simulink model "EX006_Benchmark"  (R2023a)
settings: Solver=ode23tb  StartTime=0.0  StopTime=20e3  MaxStep=1e-1  RelTol=1e-4
undefined symbols (not defined in the file or in its folder): anodeSupplyPressure
libraries: component_lib x38, slpidlib x5, simulink x1, base_lib x1

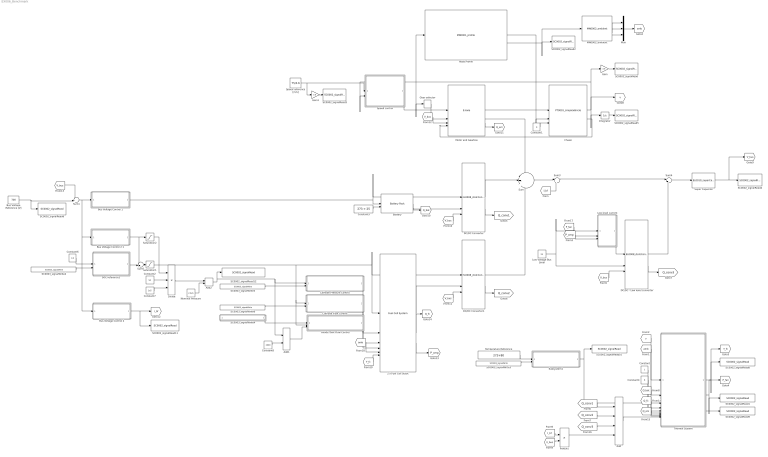
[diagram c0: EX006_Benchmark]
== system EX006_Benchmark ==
  2 x Fuel Cell Stack : component_lib/Fuel Cell System  n_st=2  n=375
  Add : Sum  Inputs=++++
  Add1 : Sum
  Add2 : Sum
  Anode Tank Flow Control : Subsystem  mask{n_cell=375}
      mask prompts: n_cell "Cells [-]"
  Battery : component_lib/Battery Pack  SOC_0=0.5  Nx=120  Ny=180
  Bus Voltage Control 1 : Subsystem
  Bus Voltage Control 2 : Subsystem
  Bus Voltage Control 2 1 : Subsystem
  Bus Voltage Reference [V] : Constant  Value=700
  Cathode Flow Control : Subsystem  mask{lambda_O2_ref=2, n_cell=375}
      mask prompts: lambda_O2_ref "Oxygen stoich. reference [-]:"; n_cell "Cells [-]:"
  Cathode Pressure Control : Subsystem
  Chassi : component_lib/Powertrain/PT0001_simpleVehicle  m=40e3  r_w=0.5  A_f=10  C_d=0.5  rho_air=1.225  c_r0=0.0060  c_r1=2.3e-7  gain=600  v0=75/3.6  x0=0
  Constant : Constant
  Constant1 : Constant  Value=0
  Constant2 : Constant  Value=50
  Constant3 : Constant  Value=273 + 25
  Constant4 : Constant  Value=8
  Constant6 : Constant  Value=0.5
  Constant7 : Constant  Value=1e5
  Constant8 : Constant  Value=2000
  DC/DC - Low level converter : component_lib/Electrochemistry/EL0008_dcdcConverter  eta_up=0.99  eta_down=0.99
  DC/DC Converter : component_lib/Electrochemistry/EL0008_dcdcConverter  eta_up=0.99  eta_down=0.99
  DC/DC Converter1 : component_lib/Electrochemistry/EL0008_dcdcConverter  eta_up=0.99  eta_down=0.99
  Divide : Product  Inputs=*/*
  Gain : Gain  Gain=3.6
  Gain1 : Gain  Gain=3.6
  Gear selector : Relay  OnSwitchValue=22  OffSwitchValue=21.5  OnOutputValue=4  OffOutputValue=3
  Integrator : Integrator
  Low Voltage Bus Level : Constant  Value=24
  Low level current : Subsystem
  MN0002_ambient : component_lib/Mission/MN0002_ambient  p_0=1.01e5  T_0=273 + 20  RH_0=0.2
  Motor and Gearbox : component_lib/E-Axle  n=3  V_nom=700
  Mux : Mux  Inputs=3
  Nominal Pressure : Constant  Value=2.5e5
  Product : Product
  Road Profile : component_lib/Mission/MN0001_profile  profile=Sodertalje_Norrkoping.mat  x0=0  N_lookahead=100
  SC0002_signalRead : component_lib/Data & Control/SC0002_signalRead  SigName=velocity
  SC0002_signalRead1 : component_lib/Data & Control/SC0002_signalRead  SigName=fanPower
  SC0002_signalRead10 : component_lib/Data & Control/SC0002_signalRead  SigName=coolantValve
  SC0002_signalRead11 : component_lib/Data & Control/SC0002_signalRead  SigName=burnoffCurrent
  SC0002_signalRead12 : component_lib/Data & Control/SC0002_signalRead  SigName=pressureReference
  SC0002_signalRead2 : component_lib/Data & Control/SC0002_signalRead  SigName=altitude
  SC0002_signalRead3 : component_lib/Data & Control/SC0002_signalRead  SigName=velocityReference
  SC0002_signalRead4 : component_lib/Data & Control/SC0002_signalRead  SigName=busVoltage
  SC0002_signalRead5 : component_lib/Data & Control/SC0002_signalRead  SigName=distance
  SC0002_signalRead6 : component_lib/Data & Control/SC0002_signalRead  SigName=busVoltageReference
  SC0002_signalRead8 : component_lib/Data & Control/SC0002_signalRead  SigName=fuelCellTemperature
  SC0002_signalRead9 : component_lib/Data & Control/SC0002_signalRead  SigName=motorTemperature
  SC0003_signalWrite2 : component_lib/Data & Control/SC0003_signalWrite  SigName=stateOfCharge
  SC0003_signalWrite3 : component_lib/Data & Control/SC0003_signalWrite  SigName=fuelCellTemperature
  SC0003_signalWrite4 : Subsystem  AncestorBlock=component_lib/Data & Control/SC0003_signalWrite  mask{SigName=anodeSupplyPressure}
      mask prompts: SigName "Signal identifier:"
      mask init:
      | % set signal name in goto tag
      | set_param([gcb, '/', 'From'], 'GotoTag', SigName)
  SC0003_signalWrite5 : component_lib/Data & Control/SC0003_signalWrite  SigName=cathodeSupplyPressure
  SC0003_signalWrite6 : component_lib/Data & Control/SC0003_signalWrite  SigName=compressorFlow
  SOC-reference1 : Subsystem
  Saturation1 : Saturate  UpperLimit=600  LowerLimit=20
  Saturation2 : Saturate  UpperLimit=50  LowerLimit=0
  Speed control : Subsystem
  Speed reference [m/s] : Constant  Value=75/3.6
  Subsystem1 : Subsystem
  Sum : Sum  Inputs=-++
  Sum1 : Sum  Inputs=-+|
  Sum3 : Sum  Inputs=|+-
  Sum4 : Sum  Inputs=|+-
  Sum5 : Sum  Inputs=++|
  Super Capacitor : component_lib/Electrochemistry/EL0010_superCapacitor  C=1  V_bus0=700
  Temperature Reference : Constant  Value=273+80
  Thermal System : Subsystem
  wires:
  Motor and Gearbox/1 -> Chassi/1
  Chassi/2 -> Motor and Gearbox/4
  Road Profile/1 -> Chassi/2
  Speed reference [m/s]/1 -> Gain1/1, Speed control/1(v_ref [m/s])
  Gear selector/1 -> Motor and Gearbox/2
  Integrator/1 -> SC0002_signalRead5/1
  Gain/1 -> SC0002_signalRead/1
  Road Profile/2 -> MN0002_ambient/1, SC0002_signalRead2/1
  Gain1/1 -> SC0002_signalRead3/1
  Super Capacitor/1 -> SC0002_signalRead4/1, [V_bus]
  Constant1/1 -> Chassi/3
  Battery/1 -> DC/DC Converter/2
  DC/DC Converter/1 -> Sum/2
  Motor and Gearbox/2 -> Sum/1
  Bus Voltage Control 1/1(I_bat [-]) -> DC/DC Converter/1, Battery/1
  DC/DC Converter1/1 -> Sum/3
  Bus Voltage Reference [V]/1 -> Sum1/2, SC0002_signalRead6/1
  Sum/1 -> Sum3/1
  [I_bf] -> Sum3/2
  MN0002_ambient/3 -> Mux/3
  MN0002_ambient/1 -> Mux/1
  MN0002_ambient/2 -> Mux/2
  Mux/1 -> [amb]
  Sum3/1 -> Sum4/1
  Thermal System/2(P_fan [J/s]) -> [P_fan], SC0002_signalRead1/1
  Constant4/1 -> Thermal System/5(W_pump [kg/s])
  [Q_em] -> Thermal System/8(Q_em [J/s])
  Thermal System/1(T_fc [K]) -> [T_fc], SC0002_signalRead8/1
  [Q_bat] -> Thermal System/6(Q_bat [J/s])
  Subsystem1/1(cv [-]) -> Thermal System/3(cv [-]), SC0002_signalRead10/1
  [v] -> Thermal System/1(v [m/s])
  Constant/1 -> Thermal System/4(fan [-])
  Thermal System/3(T_em [K]) -> SC0002_signalRead9/1
  [Q_fc] -> Thermal System/7(Q_fc [J/s])
  [amb] -> Thermal System/2(amb (T,p,RH))
  Low Voltage Bus Level/1 -> DC/DC - Low level converter/2, Low level current/1(V [V])
  DC/DC - Low level converter/1 -> Sum4/2
  Sum4/1 -> Super Capacitor/1
  Add/1 -> Thermal System/9(Q_elec [J/s])
  [Q_conv1] -> Add/1
  [Q_conv2] -> Add/2
  [Q_conv3] -> Add/3
  DC/DC Converter/2 -> [Q_conv1]
  DC/DC Converter1/2 -> [Q_conv2]
  DC/DC - Low level converter/2 -> [Q_conv3]
  [V_bus] -> Motor and Gearbox/3
  [V_bus] -> Sum1/1
  Battery/3 -> [Q_bat]
  [I_bf] -> Product/1
  [V_bus] -> Product/2
  Product/1 -> Add/4
  Motor and Gearbox/3 -> [Q_em]
  Temperature Reference/1 -> Subsystem1/1(T_fc_ref [K])
  Chassi/1 -> Integrator/1, [v], Gain/1, Road Profile/1, Speed control/2(v [m/s]), Gear selector/1
  SC0003_signalWrite3/1 -> Subsystem1/2(T_fc [K])
  [P_fan] -> Low level current/2(P_1 [J/s])
  Speed control/1(Tq_sig [-]) -> Motor and Gearbox/1
  Constant8/1 -> Add1/2
  [amb] -> 2 x Fuel Cell Stack/5
  Bus Voltage Control 2 1/1(I_fc+ [A]) -> Saturation2/1, Sum5/1
  Add1/1 -> Anode Tank Flow Control/3(p_ref [Pa])
  SC0003_signalWrite2/1 -> SOC-reference1/2(SOC [-])
  Divide/1 -> Add2/1
  Nominal Pressure/1 -> Add2/2
  SC0003_signalWrite4/1(y) -> Anode Tank Flow Control/1(p [Pa])
  Constant7/1 -> Divide/3
  Cathode Pressure Control/1(throttle [-]) -> 2 x Fuel Cell Stack/2
  Saturation1/1 -> Anode Tank Flow Control/2(I_fc [A]), Cathode Flow Control/1(I_fc [A]), DC/DC Converter1/1, 2 x Fuel Cell Stack/1
  SC0003_signalWrite5/1 -> Cathode Pressure Control/2(p [Pa])
  Anode Tank Flow Control/1(W_H2_tank [kg/s]) -> 2 x Fuel Cell Stack/4
  Add2/1 -> Add1/1, Cathode Pressure Control/1(p_ref [Pa]), SC0002_signalRead12/1
  Bus Voltage Control 2/1(I_bf [A]) -> SC0002_signalRead11/1, [I_bf]
  Cathode Flow Control/1(w_cmp [rad/s]) -> 2 x Fuel Cell Stack/3
  Constant2/1 -> Divide/2
  Saturation2/1 -> Divide/1
  Sum1/1 -> Bus Voltage Control 2/1(V_ref - V_bus [V]), Bus Voltage Control 2 1/1(V_ref - V_bus [V]), Bus Voltage Control 1/1(V_ref - V_bus [V])
  Sum5/1 -> Saturation1/1
  SOC-reference1/1(I_fc_nom [A]) -> Sum5/2
  Constant6/1 -> SOC-reference1/1(SOC_ref [-])
  2 x Fuel Cell Stack/3 -> [P_cmp]
  SC0003_signalWrite6/1 -> Cathode Flow Control/2(W_ca [kg/s])
  [T_fc] -> 2 x Fuel Cell Stack/6
  2 x Fuel Cell Stack/2 -> [Q_fc]
  2 x Fuel Cell Stack/1 -> DC/DC Converter1/2
  [V_bus] -> DC/DC Converter1/3
  [V_bus] -> DC/DC Converter/3
  Constant3/1 -> Battery/2
  Low level current/1(I [A]) -> DC/DC - Low level converter/1
  [P_cmp] -> Low level current/3(P_2 [J/s])
  [V_bus] -> DC/DC - Low level converter/3

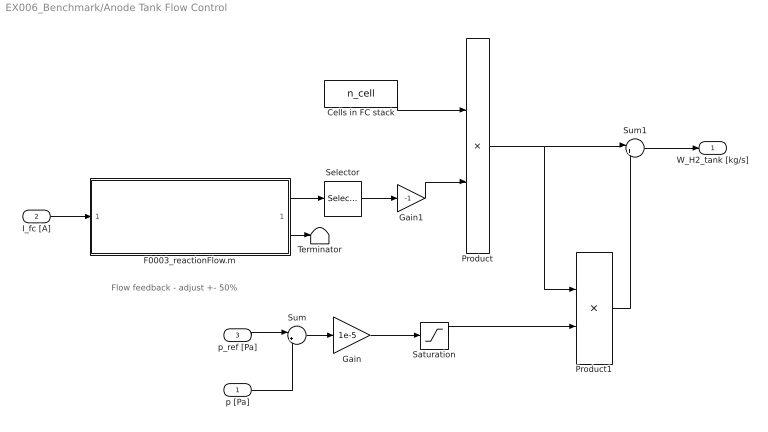
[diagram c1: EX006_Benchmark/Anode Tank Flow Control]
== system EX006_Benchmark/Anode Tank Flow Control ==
  note: Flow feedback - adjust +- 50%
  p [Pa] : Inport
  I_fc [A] : Inport  Port=2
  p_ref [Pa] : Inport  Port=3
  Cells in FC stack : Constant  Value=n_cell
  F0003_reactionFlow.m : MATLAB Function  TreatAsAtomicUnit=on
  Gain : Gain  Gain=1e-5
  Gain1 : Gain  Gain=-1
  Product : Product
  Product1 : Product
  Saturation : Saturate
  Selector : Selector  InputPortWidth=4  IndexOptions=Index vector (dialog)  Indices=1  OutputSizes=1
  Sum : Sum  Inputs=|+-
  Sum1 : Sum  Inputs=|++
  Terminator : Terminator
  W_H2_tank [kg/s] : Outport
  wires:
  Product1/1 -> Sum1/2
  Sum/1 -> Gain/1
  Sum1/1 -> W_H2_tank [kg/s]/1
  Product/1 -> Product1/1, Sum1/1
  p [Pa]/1 -> Sum/2
  p_ref [Pa]/1 -> Sum/1
  Cells in FC stack/1 -> Product/1
  F0003_reactionFlow.m/2(W_ca) -> Terminator/1
  I_fc [A]/1 -> F0003_reactionFlow.m/1(I)
  F0003_reactionFlow.m/1(W_an) -> Selector/1
  Selector/1 -> Gain1/1
  Gain1/1 -> Product/2
  Gain/1 -> Saturation/1
  Saturation/1 -> Product1/2

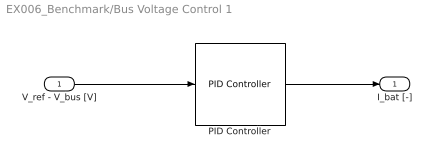
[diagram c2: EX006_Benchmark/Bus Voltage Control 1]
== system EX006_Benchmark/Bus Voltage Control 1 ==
  V_ref - V_bus [V] : Inport
  PID Controller : slpidlib/PID Controller  Controller=PID  Form=Parallel  TimeDomain=Continuous-time  UseExternalTs=off  SampleTime=-1  IntegratorMethod=Forward Euler  FilterMethod=Forward Euler  ControllerParametersSource=internal  P=1e2  I=1  UseKiTs=off  D=0  N=100  UseFilter=on  TunerSelectOption=Transfer Function Based (PID Tuner App)  ZeroCross=off  InitialConditionSource=internal  InitialConditionForIntegrator=0  InitialConditionForFilter=0  DifferentiatorICPrevScaledInput=0  ExternalReset=none  TrackingMode=off  Kt=1  LimitOutput=on  SatLimitsSource=internal  UpperSaturationLimit=350  LowerSaturationLimit=-350  LinearizeAsGain=on  AntiWindupMode=clamping  Kb=1  LimitIntegrator=off  UpperIntegratorSaturationLimit=inf  LowerIntegratorSaturationLimit=-inf  POutMin=[]  POutMax=[]  IOutMin=[]  IOutMax=[]  DOutMin=[]  DOutMax=[]  NOutMin=[]  NOutMax=[]  SumOutMin=[]  SumOutMax=[]  SaturationOutMin=[]  SaturationOutMax=[]  PParamMin=[]  PParamMax=[]  IParamMin=[]  IParamMax=[]  DParamMin=[]  DParamMax=[]  NParamMin=[]  NParamMax=[]  KbParamMin=[]  KbParamMax=[]  KtParamMin=[]  KtParamMax=[]  KbOutMin=[]  KbOutMax=[]  KtOutMin=[]  KtOutMax=[]  IntegratorOutMin=[]  IntegratorOutMax=[]  FilterOutMin=[]  FilterOutMax=[]  SumI1OutMin=[]  SumI1OutMax=[]  SumI2OutMin=[]  SumI2OutMax=[]  SumI3OutMin=[]  SumI3OutMax=[]  SumI4OutMin=[]  SumI4OutMax=[]  SumDOutMin=[]  SumDOutMax=[]  DifferentiatorOutMin=[]  DifferentiatorOutMax=[]  FilterDiffOutCoefMin=[]  FilterDiffOutCoefMax=[]  ReciprocalOutMin=[]  ReciprocalOutMax=[]  SumDenOutMin=[]  SumDenOutMax=[]  SumNumOutMin=[]  SumNumOutMax=[]  DivideOutMin=[]  DivideOutMax=[]  UdiffTsProdOutMin=[]  UdiffTsProdOutMax=[]  NTsProdOutMin=[]  NTsProdOutMax=[]  UintegralTsProdOutMin=[]  UintegralTsProdOutMax=[]  UngainTsProdOutMin=[]  UngainTsProdOutMax=[]  ClampingZeroOutDataTypeStr=Inherit: Inherit via back propagation  ClampingZeroOutMin=[]  ClampingZeroOutMax=[]  FilterDenConstantOutDataTypeStr=Inherit: Inherit via back propagation  FilterDenConstantOutMin=[]  FilterDenConstantOutMax=[]  PCopyOutDataTypeStr=Inherit: Inherit via back propagation  PCopyOutMin=[]  PCopyOutMax=[]  NCopyOutDataTypeStr=Inherit: Inherit via back propagation  NCopyOutMin=[]  NCopyOutMax=[]  IntegratorContinuousStateAttributes=''  IntegratorStateMustResolveToSignalObject=off  IntegratorRTWStateStorageClass=Auto  FilterContinuousStateAttributes=''  FilterStateMustResolveToSignalObject=off  FilterRTWStateStorageClass=Auto  ParallelPVariant=InternalParameters  IdealPVariant=Disabled  IVariant=InternalParameters  DVariant=InternalParameters  IntegratorVariant=Continuous  SatVariant=Enabled  AWVariant=ContClampingParallel  PCopyVariant=Disabled  TRVariant=Disabled  FdbkBlocksVariant=Forward  IdealPFdbkVariant=Disabled  SatFdbkVariant=Disabled  DerivativeFilterVariant=ContFilter  NVariant=InternalParameters  NCopyVariant=Disabled  FilterICVariant=InternalICsFilter  IntegratorICVariant=InternalICs  ExternalResetVariant=Disabled  TRSumVariant=Passthrough  SumFdbkVariant=Disabled  SumVariant=Sum_PID  TsampFilterVariant=InternalTs  TsampNgainVariant=Passthrough  TsampIntegralVariant=Disabled_SignalSpec  ExternalSaturationOutDataTypeStr=Inherit: Same as second input
  I_bat [-] : Outport
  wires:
  PID Controller/1 -> I_bat [-]/1
  V_ref - V_bus [V]/1 -> PID Controller/1

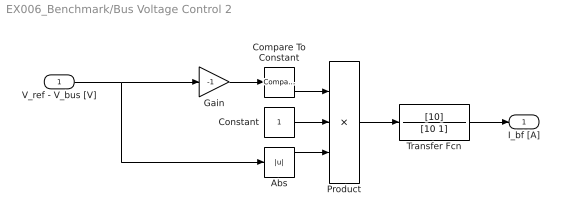
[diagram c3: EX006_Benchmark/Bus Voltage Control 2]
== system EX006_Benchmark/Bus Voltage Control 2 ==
  V_ref - V_bus [V] : Inport
  Abs : Abs
  Compare To Constant : simulink/Logic and Bit Operations/Compare To Constant  relop=>=  const=10  OutDataTypeStr=boolean
  Constant : Constant
  Gain : Gain  Gain=-1
  Product : Product  Inputs=3
  Transfer Fcn : TransferFcn  Numerator=[10]  Denominator=[10 1]
  I_bf [A] : Outport
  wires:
  Gain/1 -> Compare To Constant/1
  Transfer Fcn/1 -> I_bf [A]/1
  Compare To Constant/1 -> Product/1
  Product/1 -> Transfer Fcn/1
  V_ref - V_bus [V]/1 -> Abs/1, Gain/1
  Abs/1 -> Product/3
  Constant/1 -> Product/2

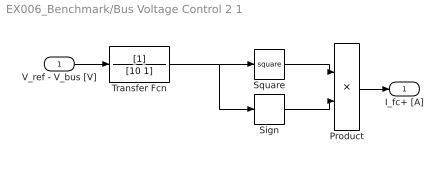
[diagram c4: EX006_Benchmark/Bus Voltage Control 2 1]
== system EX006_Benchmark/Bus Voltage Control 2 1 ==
  V_ref - V_bus [V] : Inport
  Product : Product
  Sign : Signum
  Square : Math  Operator=square
  Transfer Fcn : TransferFcn  Denominator=[10 1]
  I_fc+ [A] : Outport
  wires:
  Sign/1 -> Product/2
  Transfer Fcn/1 -> Sign/1, Square/1
  Square/1 -> Product/1
  V_ref - V_bus [V]/1 -> Transfer Fcn/1
  Product/1 -> I_fc+ [A]/1

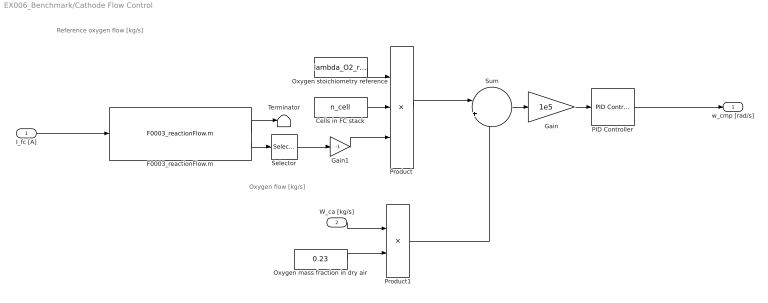
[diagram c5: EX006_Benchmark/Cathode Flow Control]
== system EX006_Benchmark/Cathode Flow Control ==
  note: Reference oxygen flow [kg/s]
  note: Oxygen flow [kg/s]
  I_fc [A] : Inport
  W_ca [kg/s] : Inport  Port=2
  Cells in FC stack : Constant  Value=n_cell
  F0003_reactionFlow.m : base_lib/F0003_pukrushpan2004/F0003_reactionFlow.m  SystemSampleTime=-1  VariantActivationTime=update diagram  Latency=0  AutoFrameSizeCalculation=off
  Gain : Gain  Gain=1e5
  Gain1 : Gain  Gain=-1
  Oxygen mass fraction in dry air : Constant  Value=0.23
  Oxygen stoichiometry reference : Constant  Value=lambda_O2_ref
  PID Controller : slpidlib/PID Controller  Controller=PID  Form=Parallel  TimeDomain=Continuous-time  UseExternalTs=off  SampleTime=-1  IntegratorMethod=Forward Euler  FilterMethod=Forward Euler  ControllerParametersSource=internal  P=30  I=0.7  UseKiTs=off  D=0  N=100  UseFilter=on  TunerSelectOption=Transfer Function Based (PID Tuner App)  ZeroCross=off  InitialConditionSource=internal  InitialConditionForIntegrator=10e3  InitialConditionForFilter=10e3  DifferentiatorICPrevScaledInput=0  ExternalReset=none  TrackingMode=off  Kt=1  LimitOutput=on  SatLimitsSource=internal  UpperSaturationLimit=20e3  LowerSaturationLimit=3e3  LinearizeAsGain=on  AntiWindupMode=clamping  Kb=1e-1  LimitIntegrator=off  UpperIntegratorSaturationLimit=inf  LowerIntegratorSaturationLimit=-inf  POutMin=[]  POutMax=[]  IOutMin=[]  IOutMax=[]  DOutMin=[]  DOutMax=[]  NOutMin=[]  NOutMax=[]  SumOutMin=[]  SumOutMax=[]  SaturationOutMin=[]  SaturationOutMax=[]  PParamMin=[]  PParamMax=[]  IParamMin=[]  IParamMax=[]  DParamMin=[]  DParamMax=[]  NParamMin=[]  NParamMax=[]  KbParamMin=[]  KbParamMax=[]  KtParamMin=[]  KtParamMax=[]  KbOutMin=[]  KbOutMax=[]  KtOutMin=[]  KtOutMax=[]  IntegratorOutMin=[]  IntegratorOutMax=[]  FilterOutMin=[]  FilterOutMax=[]  SumI1OutMin=[]  SumI1OutMax=[]  SumI2OutMin=[]  SumI2OutMax=[]  SumI3OutMin=[]  SumI3OutMax=[]  SumI4OutMin=[]  SumI4OutMax=[]  SumDOutMin=[]  SumDOutMax=[]  DifferentiatorOutMin=[]  DifferentiatorOutMax=[]  FilterDiffOutCoefMin=[]  FilterDiffOutCoefMax=[]  ReciprocalOutMin=[]  ReciprocalOutMax=[]  SumDenOutMin=[]  SumDenOutMax=[]  SumNumOutMin=[]  SumNumOutMax=[]  DivideOutMin=[]  DivideOutMax=[]  UdiffTsProdOutMin=[]  UdiffTsProdOutMax=[]  NTsProdOutMin=[]  NTsProdOutMax=[]  UintegralTsProdOutMin=[]  UintegralTsProdOutMax=[]  UngainTsProdOutMin=[]  UngainTsProdOutMax=[]  ClampingZeroOutDataTypeStr=Inherit: Inherit via back propagation  ClampingZeroOutMin=[]  ClampingZeroOutMax=[]  FilterDenConstantOutDataTypeStr=Inherit: Inherit via back propagation  FilterDenConstantOutMin=[]  FilterDenConstantOutMax=[]  PCopyOutDataTypeStr=Inherit: Inherit via back propagation  PCopyOutMin=[]  PCopyOutMax=[]  NCopyOutDataTypeStr=Inherit: Inherit via back propagation  NCopyOutMin=[]  NCopyOutMax=[]  IntegratorContinuousStateAttributes=''  IntegratorStateMustResolveToSignalObject=off  IntegratorRTWStateStorageClass=Auto  FilterContinuousStateAttributes=''  FilterStateMustResolveToSignalObject=off  FilterRTWStateStorageClass=Auto  ParallelPVariant=InternalParameters  IdealPVariant=Disabled  IVariant=InternalParameters  DVariant=InternalParameters  IntegratorVariant=Continuous  SatVariant=Enabled  AWVariant=ContClampingParallel  PCopyVariant=Disabled  TRVariant=Disabled  FdbkBlocksVariant=Forward  IdealPFdbkVariant=Disabled  SatFdbkVariant=Disabled  DerivativeFilterVariant=ContFilter  NVariant=InternalParameters  NCopyVariant=Disabled  FilterICVariant=InternalICsFilter  IntegratorICVariant=InternalICs  ExternalResetVariant=Disabled  TRSumVariant=Passthrough  SumFdbkVariant=Disabled  SumVariant=Sum_PID  TsampFilterVariant=InternalTs  TsampNgainVariant=Passthrough  TsampIntegralVariant=Disabled_SignalSpec  ExternalSaturationOutDataTypeStr=Inherit: Same as second input
  Product : Product  Inputs=3
  Product1 : Product
  Selector : Selector  InputPortWidth=4  IndexOptions=Index vector (dialog)  Indices=2  OutputSizes=1
  Sum : Sum  Inputs=|+-
  Terminator : Terminator
  w_cmp [rad/s] : Outport
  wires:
  W_ca [kg/s]/1 -> Product1/1
  I_fc [A]/1 -> F0003_reactionFlow.m/1
  Gain/1 -> PID Controller/1
  PID Controller/1 -> w_cmp [rad/s]/1
  Sum/1 -> Gain/1
  Product1/1 -> Sum/2
  Product/1 -> Sum/1
  Cells in FC stack/1 -> Product/2
  Gain1/1 -> Product/3
  F0003_reactionFlow.m/1 -> Terminator/1
  Oxygen mass fraction in dry air/1 -> Product1/2
  Selector/1 -> Gain1/1
  Oxygen stoichiometry reference/1 -> Product/1
  F0003_reactionFlow.m/2 -> Selector/1

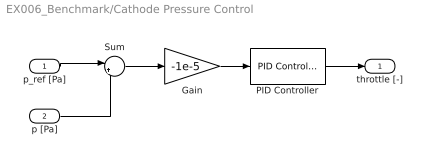
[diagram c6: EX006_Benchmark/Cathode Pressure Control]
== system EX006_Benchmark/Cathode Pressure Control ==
  p_ref [Pa] : Inport
  p [Pa] : Inport  Port=2
  Gain : Gain  Gain=-1e-5
  PID Controller : slpidlib/PID Controller  Controller=PID  Form=Parallel  TimeDomain=Continuous-time  UseExternalTs=off  SampleTime=-1  IntegratorMethod=Forward Euler  FilterMethod=Forward Euler  ControllerParametersSource=internal  P=1  I=1e-1  UseKiTs=off  D=0  N=100  UseFilter=on  TunerSelectOption=Transfer Function Based (PID Tuner App)  ZeroCross=off  InitialConditionSource=internal  InitialConditionForIntegrator=0.5  InitialConditionForFilter=0.5  DifferentiatorICPrevScaledInput=0  ExternalReset=none  TrackingMode=off  Kt=1  LimitOutput=on  SatLimitsSource=internal  UpperSaturationLimit=0.99  LowerSaturationLimit=0.01  LinearizeAsGain=on  AntiWindupMode=clamping  Kb=1  LimitIntegrator=off  UpperIntegratorSaturationLimit=inf  LowerIntegratorSaturationLimit=-inf  POutMin=[]  POutMax=[]  IOutMin=[]  IOutMax=[]  DOutMin=[]  DOutMax=[]  NOutMin=[]  NOutMax=[]  SumOutMin=[]  SumOutMax=[]  SaturationOutMin=[]  SaturationOutMax=[]  PParamMin=[]  PParamMax=[]  IParamMin=[]  IParamMax=[]  DParamMin=[]  DParamMax=[]  NParamMin=[]  NParamMax=[]  KbParamMin=[]  KbParamMax=[]  KtParamMin=[]  KtParamMax=[]  KbOutMin=[]  KbOutMax=[]  KtOutMin=[]  KtOutMax=[]  IntegratorOutMin=[]  IntegratorOutMax=[]  FilterOutMin=[]  FilterOutMax=[]  SumI1OutMin=[]  SumI1OutMax=[]  SumI2OutMin=[]  SumI2OutMax=[]  SumI3OutMin=[]  SumI3OutMax=[]  SumI4OutMin=[]  SumI4OutMax=[]  SumDOutMin=[]  SumDOutMax=[]  DifferentiatorOutMin=[]  DifferentiatorOutMax=[]  FilterDiffOutCoefMin=[]  FilterDiffOutCoefMax=[]  ReciprocalOutMin=[]  ReciprocalOutMax=[]  SumDenOutMin=[]  SumDenOutMax=[]  SumNumOutMin=[]  SumNumOutMax=[]  DivideOutMin=[]  DivideOutMax=[]  UdiffTsProdOutMin=[]  UdiffTsProdOutMax=[]  NTsProdOutMin=[]  NTsProdOutMax=[]  UintegralTsProdOutMin=[]  UintegralTsProdOutMax=[]  UngainTsProdOutMin=[]  UngainTsProdOutMax=[]  ClampingZeroOutDataTypeStr=Inherit: Inherit via back propagation  ClampingZeroOutMin=[]  ClampingZeroOutMax=[]  FilterDenConstantOutDataTypeStr=Inherit: Inherit via back propagation  FilterDenConstantOutMin=[]  FilterDenConstantOutMax=[]  PCopyOutDataTypeStr=Inherit: Inherit via back propagation  PCopyOutMin=[]  PCopyOutMax=[]  NCopyOutDataTypeStr=Inherit: Inherit via back propagation  NCopyOutMin=[]  NCopyOutMax=[]  IntegratorContinuousStateAttributes=''  IntegratorStateMustResolveToSignalObject=off  IntegratorRTWStateStorageClass=Auto  FilterContinuousStateAttributes=''  FilterStateMustResolveToSignalObject=off  FilterRTWStateStorageClass=Auto  ParallelPVariant=InternalParameters  IdealPVariant=Disabled  IVariant=InternalParameters  DVariant=InternalParameters  IntegratorVariant=Continuous  SatVariant=Enabled  AWVariant=ContClampingParallel  PCopyVariant=Disabled  TRVariant=Disabled  FdbkBlocksVariant=Forward  IdealPFdbkVariant=Disabled  SatFdbkVariant=Disabled  DerivativeFilterVariant=ContFilter  NVariant=InternalParameters  NCopyVariant=Disabled  FilterICVariant=InternalICsFilter  IntegratorICVariant=InternalICs  ExternalResetVariant=Disabled  TRSumVariant=Passthrough  SumFdbkVariant=Disabled  SumVariant=Sum_PID  TsampFilterVariant=InternalTs  TsampNgainVariant=Passthrough  TsampIntegralVariant=Disabled_SignalSpec  ExternalSaturationOutDataTypeStr=Inherit: Same as second input
  Sum : Sum  Inputs=|+-
  throttle [-] : Outport
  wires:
  Sum/1 -> Gain/1
  p [Pa]/1 -> Sum/2
  Gain/1 -> PID Controller/1
  PID Controller/1 -> throttle [-]/1
  p_ref [Pa]/1 -> Sum/1

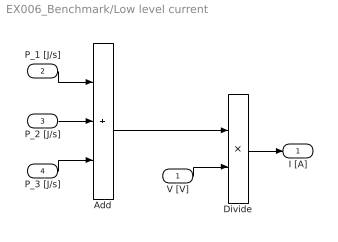
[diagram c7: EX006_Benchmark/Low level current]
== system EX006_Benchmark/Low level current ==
  V [V] : Inport
  P_1 [J/s] : Inport  Port=2
  P_2 [J/s] : Inport  Port=3
  P_3 [J/s] : Inport  Port=4
  Add : Sum  Inputs=+++
  Divide : Product  Inputs=*/
  I [A] : Outport
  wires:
  Add/1 -> Divide/1
  P_1 [J/s]/1 -> Add/1
  V [V]/1 -> Divide/2
  P_3 [J/s]/1 -> Add/3
  P_2 [J/s]/1 -> Add/2
  Divide/1 -> I [A]/1

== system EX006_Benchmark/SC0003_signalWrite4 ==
  y : Outport
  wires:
  [anodeSupplyPressure] -> y/1

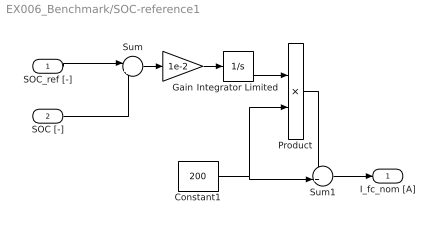
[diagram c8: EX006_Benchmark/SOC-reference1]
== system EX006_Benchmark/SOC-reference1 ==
  SOC_ref [-] : Inport
  SOC [-] : Inport  Port=2
  Constant1 : Constant  Value=200
  Gain : Gain  Gain=1e-2
  Integrator Limited : Integrator  LimitOutput=on  UpperSaturationLimit=1  LowerSaturationLimit=-1
  Product : Product
  Sum : Sum  Inputs=|+-
  Sum1 : Sum  Inputs=++|
  I_fc_nom [A] : Outport
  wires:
  Product/1 -> Sum1/1
  Integrator Limited/1 -> Product/1
  Sum1/1 -> I_fc_nom [A]/1
  Constant1/1 -> Sum1/2, Product/2
  Sum/1 -> Gain/1
  SOC [-]/1 -> Sum/2
  Gain/1 -> Integrator Limited/1
  SOC_ref [-]/1 -> Sum/1

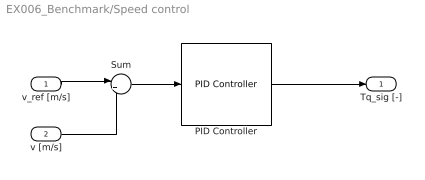
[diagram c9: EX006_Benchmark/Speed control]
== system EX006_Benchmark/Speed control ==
  v_ref [m/s] : Inport
  v [m/s] : Inport  Port=2
  PID Controller : slpidlib/PID Controller  Controller=PID  Form=Parallel  TimeDomain=Continuous-time  UseExternalTs=off  SampleTime=-1  IntegratorMethod=Forward Euler  FilterMethod=Forward Euler  ControllerParametersSource=internal  P=10  I=1e-1  UseKiTs=off  D=0  N=100  UseFilter=on  TunerSelectOption=Transfer Function Based (PID Tuner App)  ZeroCross=off  InitialConditionSource=internal  InitialConditionForIntegrator=0  InitialConditionForFilter=0  DifferentiatorICPrevScaledInput=0  ExternalReset=none  TrackingMode=off  Kt=1  LimitOutput=on  SatLimitsSource=internal  UpperSaturationLimit=1  LowerSaturationLimit=-1  LinearizeAsGain=on  AntiWindupMode=clamping  Kb=1  LimitIntegrator=off  UpperIntegratorSaturationLimit=inf  LowerIntegratorSaturationLimit=-inf  POutMin=[]  POutMax=[]  IOutMin=[]  IOutMax=[]  DOutMin=[]  DOutMax=[]  NOutMin=[]  NOutMax=[]  SumOutMin=[]  SumOutMax=[]  SaturationOutMin=[]  SaturationOutMax=[]  PParamMin=[]  PParamMax=[]  IParamMin=[]  IParamMax=[]  DParamMin=[]  DParamMax=[]  NParamMin=[]  NParamMax=[]  KbParamMin=[]  KbParamMax=[]  KtParamMin=[]  KtParamMax=[]  KbOutMin=[]  KbOutMax=[]  KtOutMin=[]  KtOutMax=[]  IntegratorOutMin=[]  IntegratorOutMax=[]  FilterOutMin=[]  FilterOutMax=[]  SumI1OutMin=[]  SumI1OutMax=[]  SumI2OutMin=[]  SumI2OutMax=[]  SumI3OutMin=[]  SumI3OutMax=[]  SumI4OutMin=[]  SumI4OutMax=[]  SumDOutMin=[]  SumDOutMax=[]  DifferentiatorOutMin=[]  DifferentiatorOutMax=[]  FilterDiffOutCoefMin=[]  FilterDiffOutCoefMax=[]  ReciprocalOutMin=[]  ReciprocalOutMax=[]  SumDenOutMin=[]  SumDenOutMax=[]  SumNumOutMin=[]  SumNumOutMax=[]  DivideOutMin=[]  DivideOutMax=[]  UdiffTsProdOutMin=[]  UdiffTsProdOutMax=[]  NTsProdOutMin=[]  NTsProdOutMax=[]  UintegralTsProdOutMin=[]  UintegralTsProdOutMax=[]  UngainTsProdOutMin=[]  UngainTsProdOutMax=[]  ClampingZeroOutDataTypeStr=Inherit: Inherit via back propagation  ClampingZeroOutMin=[]  ClampingZeroOutMax=[]  FilterDenConstantOutDataTypeStr=Inherit: Inherit via back propagation  FilterDenConstantOutMin=[]  FilterDenConstantOutMax=[]  PCopyOutDataTypeStr=Inherit: Inherit via back propagation  PCopyOutMin=[]  PCopyOutMax=[]  NCopyOutDataTypeStr=Inherit: Inherit via back propagation  NCopyOutMin=[]  NCopyOutMax=[]  IntegratorContinuousStateAttributes=''  IntegratorStateMustResolveToSignalObject=off  IntegratorRTWStateStorageClass=Auto  FilterContinuousStateAttributes=''  FilterStateMustResolveToSignalObject=off  FilterRTWStateStorageClass=Auto  ParallelPVariant=InternalParameters  IdealPVariant=Disabled  IVariant=InternalParameters  DVariant=InternalParameters  IntegratorVariant=Continuous  SatVariant=Enabled  AWVariant=ContClampingParallel  PCopyVariant=Disabled  TRVariant=Disabled  FdbkBlocksVariant=Forward  IdealPFdbkVariant=Disabled  SatFdbkVariant=Disabled  DerivativeFilterVariant=ContFilter  NVariant=InternalParameters  NCopyVariant=Disabled  FilterICVariant=InternalICsFilter  IntegratorICVariant=InternalICs  ExternalResetVariant=Disabled  TRSumVariant=Passthrough  SumFdbkVariant=Disabled  SumVariant=Sum_PID  TsampFilterVariant=InternalTs  TsampNgainVariant=Passthrough  TsampIntegralVariant=Disabled_SignalSpec  ExternalSaturationOutDataTypeStr=Inherit: Same as second input
  Sum : Sum  Inputs=|+-
  Tq_sig [-] : Outport
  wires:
  PID Controller/1 -> Tq_sig [-]/1
  Sum/1 -> PID Controller/1
  v_ref [m/s]/1 -> Sum/1
  v [m/s]/1 -> Sum/2

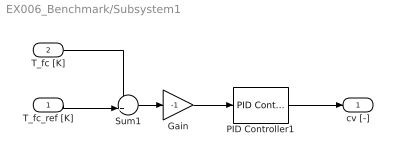
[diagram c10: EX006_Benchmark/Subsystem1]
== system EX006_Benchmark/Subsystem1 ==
  T_fc_ref [K] : Inport
  T_fc [K] : Inport  Port=2
  Gain : Gain  Gain=-1
  PID Controller1 : slpidlib/PID Controller  Controller=PID  Form=Parallel  TimeDomain=Continuous-time  UseExternalTs=off  SampleTime=-1  IntegratorMethod=Forward Euler  FilterMethod=Forward Euler  ControllerParametersSource=internal  P=1e-1  I=1e-2  UseKiTs=off  D=0  N=100  UseFilter=on  TunerSelectOption=Transfer Function Based (PID Tuner App)  ZeroCross=off  InitialConditionSource=internal  InitialConditionForIntegrator=0.5  InitialConditionForFilter=0.5  DifferentiatorICPrevScaledInput=0  ExternalReset=none  TrackingMode=off  Kt=1  LimitOutput=on  SatLimitsSource=internal  UpperSaturationLimit=0.95  LowerSaturationLimit=0.05  LinearizeAsGain=on  AntiWindupMode=clamping  Kb=1  LimitIntegrator=off  UpperIntegratorSaturationLimit=inf  LowerIntegratorSaturationLimit=-inf  POutMin=[]  POutMax=[]  IOutMin=[]  IOutMax=[]  DOutMin=[]  DOutMax=[]  NOutMin=[]  NOutMax=[]  SumOutMin=[]  SumOutMax=[]  SaturationOutMin=[]  SaturationOutMax=[]  PParamMin=[]  PParamMax=[]  IParamMin=[]  IParamMax=[]  DParamMin=[]  DParamMax=[]  NParamMin=[]  NParamMax=[]  KbParamMin=[]  KbParamMax=[]  KtParamMin=[]  KtParamMax=[]  KbOutMin=[]  KbOutMax=[]  KtOutMin=[]  KtOutMax=[]  IntegratorOutMin=[]  IntegratorOutMax=[]  FilterOutMin=[]  FilterOutMax=[]  SumI1OutMin=[]  SumI1OutMax=[]  SumI2OutMin=[]  SumI2OutMax=[]  SumI3OutMin=[]  SumI3OutMax=[]  SumI4OutMin=[]  SumI4OutMax=[]  SumDOutMin=[]  SumDOutMax=[]  DifferentiatorOutMin=[]  DifferentiatorOutMax=[]  FilterDiffOutCoefMin=[]  FilterDiffOutCoefMax=[]  ReciprocalOutMin=[]  ReciprocalOutMax=[]  SumDenOutMin=[]  SumDenOutMax=[]  SumNumOutMin=[]  SumNumOutMax=[]  DivideOutMin=[]  DivideOutMax=[]  UdiffTsProdOutMin=[]  UdiffTsProdOutMax=[]  NTsProdOutMin=[]  NTsProdOutMax=[]  UintegralTsProdOutMin=[]  UintegralTsProdOutMax=[]  UngainTsProdOutMin=[]  UngainTsProdOutMax=[]  ClampingZeroOutDataTypeStr=Inherit: Inherit via back propagation  ClampingZeroOutMin=[]  ClampingZeroOutMax=[]  FilterDenConstantOutDataTypeStr=Inherit: Inherit via back propagation  FilterDenConstantOutMin=[]  FilterDenConstantOutMax=[]  PCopyOutDataTypeStr=Inherit: Inherit via back propagation  PCopyOutMin=[]  PCopyOutMax=[]  NCopyOutDataTypeStr=Inherit: Inherit via back propagation  NCopyOutMin=[]  NCopyOutMax=[]  IntegratorContinuousStateAttributes=''  IntegratorStateMustResolveToSignalObject=off  IntegratorRTWStateStorageClass=Auto  FilterContinuousStateAttributes=''  FilterStateMustResolveToSignalObject=off  FilterRTWStateStorageClass=Auto  ParallelPVariant=InternalParameters  IdealPVariant=Disabled  IVariant=InternalParameters  DVariant=InternalParameters  IntegratorVariant=Continuous  SatVariant=Enabled  AWVariant=ContClampingParallel  PCopyVariant=Disabled  TRVariant=Disabled  FdbkBlocksVariant=Forward  IdealPFdbkVariant=Disabled  SatFdbkVariant=Disabled  DerivativeFilterVariant=ContFilter  NVariant=InternalParameters  NCopyVariant=Disabled  FilterICVariant=InternalICsFilter  IntegratorICVariant=InternalICs  ExternalResetVariant=Disabled  TRSumVariant=Passthrough  SumFdbkVariant=Disabled  SumVariant=Sum_PID  TsampFilterVariant=InternalTs  TsampNgainVariant=Passthrough  TsampIntegralVariant=Disabled_SignalSpec  ExternalSaturationOutDataTypeStr=Inherit: Same as second input
  Sum1 : Sum  Inputs=-+|
  cv [-] : Outport
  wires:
  T_fc [K]/1 -> Sum1/1
  Gain/1 -> PID Controller1/1
  Sum1/1 -> Gain/1
  PID Controller1/1 -> cv [-]/1
  T_fc_ref [K]/1 -> Sum1/2

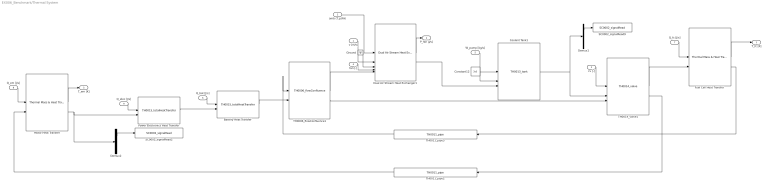
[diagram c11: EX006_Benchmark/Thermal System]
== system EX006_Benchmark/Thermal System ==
  v [m/s] : Inport
  amb (T,p,RH) : Inport  Port=2
  cv [-] : Inport  Port=3
  fan [-] : Inport  Port=4
  W_pump [kg/s] : Inport  Port=5
  Q_bat [J/s] : Inport  Port=6
  Q_fc [J/s] : Inport  Port=7
  Q_em [J/s] : Inport  Port=8
  Q_elec [J/s] : Inport  Port=9
  Battery Heat Transfer : component_lib/Thermal Systems/TH0015_totalHeatTransfer  T_max=273+100  T_min=273
  Constant12 : Constant  Value=2e5
  Coolant Tank1 : component_lib/Thermal Systems/TH0013_tank  V=5e-3  T0=273.15 + 80
  Demux1 : Demux  Outputs=3
  Demux2 : Demux  Outputs=3
  Dual Air Stream Heat Exchanger1 : component_lib/Dual Air Stream Heat Exchanger  HtH=1.1  StS=0.95
  Fuel Cell Heat Transfer : component_lib/Thermal Mass & Heat Transfer  n=375*2*10  d=2e-3  L=50e-2  m=72  cp=420  T_0=273 + 80
  Ground : Ground
  Motor Heat Transfer : component_lib/Thermal Mass & Heat Transfer  n=100*3  d=5e-3  L=30e-2  m=200  cp=420  T_0=273 + 20
  Power Electronics Heat Transfer : component_lib/Thermal Systems/TH0015_totalHeatTransfer  T_max=273+100  T_min=273
  SC0002_signalRead2 : component_lib/Data & Control/SC0002_signalRead  SigName=powerElectronicsTemperature
  SC0002_signalRead9 : component_lib/Data & Control/SC0002_signalRead  SigName=coolantTemperature
  TH0006_flowConfluence1 : component_lib/Thermal Systems/TH0006_flowConfluence  gain=0.01
  TH0011_pipe2 : component_lib/Thermal Systems/TH0011_pipe  d=3e-2  L=2  e=0.006e-3  T_0=273 + 20
  TH0011_pipe3 : component_lib/Thermal Systems/TH0011_pipe  d=3e-2  L=2  e=0.006e-3  T_0=273 + 20
  TH0014_valve1 : component_lib/Thermal Systems/TH0014_valve  d=10e-2  dr=5e-2  C_d=0.9
  T_fc [K] : Outport
  P_fan [J/s] : Outport  Port=2
  T_em [K] : Outport  Port=3
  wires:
  Demux2/1 -> SC0002_signalRead2/1
  TH0014_valve1/2 -> TH0011_pipe2/1
  Power Electronics Heat Transfer/1 -> Battery Heat Transfer/2
  cv [-]/1 -> TH0014_valve1/1
  TH0006_flowConfluence1/1 -> Dual Air Stream Heat Exchanger1/5
  TH0006_flowConfluence1/2 -> TH0014_valve1/3
  amb (T,p,RH)/1 -> Dual Air Stream Heat Exchanger1/1
  Battery Heat Transfer/1 -> TH0006_flowConfluence1/2
  Ground/1 -> Dual Air Stream Heat Exchanger1/3
  fan [-]/1 -> Dual Air Stream Heat Exchanger1/4
  Motor Heat Transfer/2 -> Power Electronics Heat Transfer/2, Demux2/1
  Fuel Cell Heat Transfer/2 -> TH0011_pipe3/1
  TH0014_valve1/1 -> Fuel Cell Heat Transfer/2
  Q_elec [J/s]/1 -> Power Electronics Heat Transfer/1
  v [m/s]/1 -> Dual Air Stream Heat Exchanger1/2
  TH0011_pipe3/1 -> TH0006_flowConfluence1/1
  TH0011_pipe2/1 -> Motor Heat Transfer/2
  Q_fc [J/s]/1 -> Fuel Cell Heat Transfer/1
  Q_em [J/s]/1 -> Motor Heat Transfer/1
  Fuel Cell Heat Transfer/1 -> T_fc [K]/1
  Dual Air Stream Heat Exchanger1/1 -> P_fan [J/s]/1
  Motor Heat Transfer/1 -> T_em [K]/1
  Q_bat [J/s]/1 -> Battery Heat Transfer/1
  Coolant Tank1/1 -> TH0014_valve1/2, Demux1/1
  Demux1/1 -> SC0002_signalRead9/1
  W_pump [kg/s]/1 -> Coolant Tank1/1
  Constant12/1 -> Coolant Tank1/2
  Dual Air Stream Heat Exchanger1/2 -> Coolant Tank1/3

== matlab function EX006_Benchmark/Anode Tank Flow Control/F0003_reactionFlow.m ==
function [W_an, W_ca] = F0003_reactionFlow(I)
% constants
F     = 96485; % [C/mol]  - Faradays constant
M_H2  = 0.002; % [kg/mol] - hydrogen molecular weight
M_O2  = 0.032; % [kg/mol] - oxygen   molecular weight
% M_N2  = 0.028; % [kg/mol] - nitrogen molecular weight
M_H2O = 0.018; % [kg/mol] - water    molecular weight

% reaction flows
W_H2_rct  = I * M_H2  /(2*F);
W_O2_rct  = I * M_O2  /(4*F);
W_H2O_rct = I * M_H2O /(2*F);

% output
W_an = [-W_H2_rct;         0;         0; 0];
W_ca = [        0; -W_O2_rct; W_H2O_rct; 0]; 
end
